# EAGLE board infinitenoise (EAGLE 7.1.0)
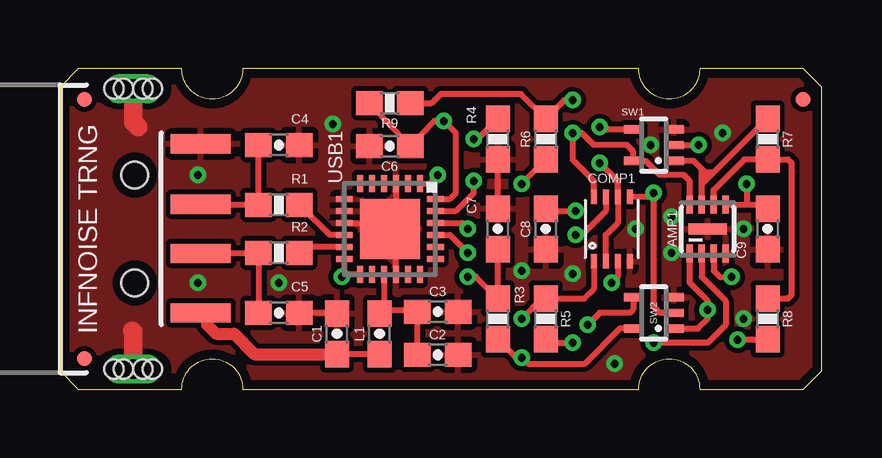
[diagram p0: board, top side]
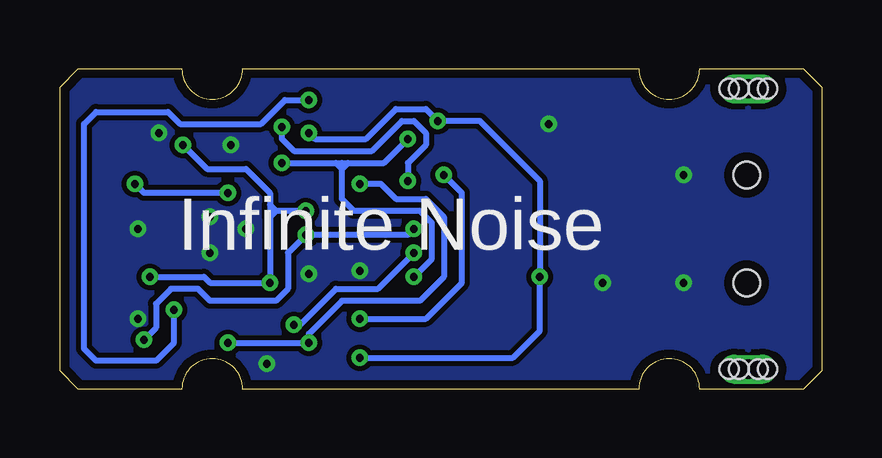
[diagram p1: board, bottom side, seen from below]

Size 31.75 x 13.36 mm. Coordinates in mm from the lower left corner, seen from the top.
Outline: 25.4,12.09 25.33,12.09
Outline: 25.4,12.09 arc90 26.67,13.36 30.99,13.36 31.75,12.6 31.75,0.76 30.99,0 26.67,0 arc90 25.4,1.27 arc90 24.13,0 7.62,0 arc90 6.35,1.27 arc90 5.08,0 0.76,0 0,0.76 0,12.6 0.76,13.36 5.08,13.36 arc90 6.35,12.09 arc90 7.62,13.36 24.13,13.36 arc90 25.4,12.09
Copper layers (1*16): Top 0.0356mm / dielectric 1.5011mm / Bottom 0.0356mm
Design rules "default *": minimum track width 8mil, minimum drill 13mil, track to track 8mil, track to pad 8mil, pad to pad 8mil, via to via 8mil, smd to smd 8mil, copper to edge 15mil, drill to drill 8mil, minimum pad ring 7mil, minimum via ring 7mil, stop-mask expansion 25mil, vias tented up to drill 14mil, thermal gap 10mil

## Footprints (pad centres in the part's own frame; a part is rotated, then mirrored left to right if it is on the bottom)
DFN6-2X3 = smd 0.28 x 0.75: 1 -0.75,-1.025; 2 -0.25,-1.025; 3 0.25,-1.025; 4 0.75,-1.025; 5 0.75,1.025; 6 0.25,1.025; 7 -0.25,1.025; 8 -0.75,1.025 | smd 1.6 x 0.45: EXP 0,0
0603-CAP = smd 1.1 x 1: 1 -0.85,0; 2 0.85,0
SSOP8-P-0.50A = smd 0.25 x 0.6: 1 -0.75,-1.35; 2 -0.25,-1.35; 3 0.25,-1.35; 4 0.75,-1.35; 5 0.75,1.35; 6 0.25,1.35; 7 -0.25,1.35; 8 -0.75,1.35
MICRO-FIDUCIAL = smd 0.635 x 0.635: 1 0,0
0603-IND = smd 1.1 x 1: 1 -0.85,0; 2 0.85,0
0603-RES = smd 1.1 x 1: 1 -0.85,0; 2 0.85,0
SC70-5L = smd 0.35 x 0.8: 1 -0.65,-0.85; 2 0,-0.85; 3 0.65,-0.85; 4 0.65,0.85; 5 -0.65,0.85
QFN24-4X4 = smd 0.7 x 0.25: 1 -1.9,1.25; 2 -1.9,0.75; 3 -1.9,0.25; 4 -1.9,-0.25; 5 -1.9,-0.75; 6 -1.9,-1.25; 13 1.9,-1.25; 14 1.9,-0.75; 15 1.9,-0.25; 16 1.9,0.25; 17 1.9,0.75; 18 1.9,1.25 | smd 0.25 x 0.7: 7 -1.25,-1.9; 8 -0.75,-1.9; 9 -0.25,-1.9; 10 0.25,-1.9; 11 0.75,-1.9; 12 1.25,-1.9; 19 1.25,1.9; 20 0.75,1.9; 21 0.25,1.9; 22 -0.25,1.9; 23 -0.75,1.9; 24 -1.25,1.9 | smd 2.5 x 2.5: EXP 0,0
USB-A-SMT-MALE = smd 0.8 x 2.5: 1 -3.5,-5.87; 2 -1.027,-5.87; 3 1.027,-5.87; 4 3.551,-5.87 | drill 0.8 pad 0.94 long: P$1 5.85,-3.05; P$3 -5.85,-3.05 | hole 1.1: 2.25,-3.12; -2.25,-3.12 | hole 0.8: -5.85,-3.45; -5.85,-3.85; -5.85,-2.65; -5.85,-2.25; 5.85,-3.45; 5.85,-3.85; 5.85,-2.65; 5.85,-2.25

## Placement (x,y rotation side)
AMP1  TSV912IQ2T  [DFN6-2X3]  27,6.68 0 top
C1  10nF  [0603-CAP]  11.55,2.31 90 top
C2  4.7uF  [0603-CAP]  15.75,1.43 0 top
C3  100nF  [0603-CAP]  15.75,3.23 0 top
C4  47pF  [0603-CAP]  9.12,10.18 0 top
C5  47pF  [0603-CAP]  9.12,3.18 0 top
C6  100nF  [0603-CAP]  13.75,10.13 180 top
C7  10nF  [0603-CAP]  18.25,6.68 90 top
C8  220pF  [0603-CAP]  20.25,6.68 90 top
C9  220pF  [0603-CAP]  29.5,6.68 90 top
COMP1  TC75W57FK  [SSOP8-P-0.50A]  23,6.68 0 top
FID1  FIDUCIALUFIDUCIAL  [MICRO-FIDUCIAL]  1.02,1.27 0 top
FID2  FIDUCIALUFIDUCIAL  [MICRO-FIDUCIAL]  1.02,12.09 0 top
FID3  FIDUCIALUFIDUCIAL  [MICRO-FIDUCIAL]  30.99,12.09 0 top
L1  FERRITE-BEAD0603-IND  [0603-IND]  13.32,2.31 90 top
R1  27  [0603-RES]  9.12,7.68 0 top
R2  27  [0603-RES]  9.12,5.68 0 top
R3  10K  [0603-RES]  18.25,2.93 90 top
R4  10K  [0603-RES]  18.25,10.43 90 top
R5  10K  [0603-RES]  20.25,2.93 270 top
R6  8.2K  [0603-RES]  20.25,10.43 90 top
R7  8.2K  [0603-RES]  29.5,10.43 270 top
R8  10K  [0603-RES]  29.5,2.93 270 top
R9  10K  [0603-RES]  13.75,11.93 180 top
SW1  MC74VHC1G66DFT1G  [SC70-5L]  24.75,10.18 90 top
SW2  MC74VHC1G66DFT1G  [SC70-5L]  24.75,3.18 90 top
USB1  FT240XQ  [QFN24-4X4]  13.75,6.68 270 top
X1  USBSMT-MALE  [USB-A-SMT-MALE]  0,6.68 90 top

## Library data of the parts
AMP1 C1-C9 COMP1 L1 R1-R9 SW1 SW2 USB1 X1 = infnoise
FID1-FID3 = SparkFun-Aesthetics

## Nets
A: AMP1.3 C8.2 COMP1.3 SW1.2
AMP1OUT: AMP1.1 R6.2 R9.1 SW2.1
AMP2OUT: AMP1.7 R7.1 SW1.1
B: AMP1.5 C9.2 COMP1.5 SW2.2
COMP1: COMP1.1 R5.1 USB1.1
COMP2: COMP1.7 R8.2 USB1.22
FB1: AMP1.2 R5.2 R6.1
FB2: AMP1.6 R7.2 R8.1
GND: AMP1.4 AMP1.EXP C1.2 C2.2 C3.2 C4.2 C5.2 C6.2 C7.2 C8.1 C9.1 COMP1.4 R4.1 SW1.3 SW2.3 USB1.3 USB1.7 USB1.8 USB1.9 USB1.16 USB1.EXP X1.4 X1.P$1 X1.P$3
N$2: R1.2 USB1.10
SW1EN: SW1.4 USB1.23
SW2EN: SW2.4 USB1.21
USB_M: C5.1 R2.1 X1.2
USB_P: C4.1 R1.1 X1.3
USBDM: R2.2 USB1.11
VCC: C2.1 C3.1 L1.2 USB1.15
VCC33: AMP1.8 C6.1 COMP1.8 R3.1 R9.2 SW1.5 SW2.5 USB1.12 USB1.13 USB1.24
VCCIN: C1.1 L1.1 X1.1
VREF: C7.1 COMP1.2 COMP1.6 R3.2 R4.2

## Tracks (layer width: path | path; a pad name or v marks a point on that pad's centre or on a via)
A  (via drill 0.33)
  Top 0.254: AMP1.3 27.25,4.93 27.5,4.68 v28,4.68 | SW1.2 v26.62,10.18 | COMP1.3 23.25,4.68 v23,4.43 | C8.2 20.35,7.43 v21.5,7.43
  Bottom 0.254: v26.62,10.18 25.62,9.18 24,9.18 23,8.18 23,7.68 | 23,7.68 23,7.43 | 23,7.43 23,7.18 | 23,7.18 v23,4.43 25.5,4.43 25.75,4.68 v28,4.68 | v21.5,7.43 22.75,7.43 | 22.75,7.43 23,7.43 | 22.75,7.43 23,7.68 | 22.75,7.43 23,7.18
AMP1OUT  (via drill 0.33)
  Top 0.254: SW2.1 26.6,2.53 27,2.93 v27,3.31 27,3.68 26.25,4.43 AMP1.1 | R9.1 15.5,11.93 15.88,12.3 19.23,12.3 R6.2 21.02,12.05 v21.38,12.05
  Bottom 0.254: v27,3.31 27,1.93 27.75,1.18 30.25,1.18 30.75,1.68 30.75,11.05 30.25,11.55 27.25,11.55 26.75,11.05 23.38,11.05 22.38,12.05 v21.38,12.05
AMP2OUT
  Top 0.254: AMP1.7 26.75,8.55 | 26.75,8.55 26.75,8.68 | 26.75,8.68 26.75,8.93 | 26.75,8.93 26.75,9.18 | 27.25,9.05 29.5,11.3 R7.1 | 27.25,9.05 27.12,8.93 | SW1.1 26.4,9.53 26.75,9.18 | 27.12,8.93 27,8.93 | 27,8.93 26.75,8.93 | 26.75,9.18 26.88,9.05 | 26.88,9.05 27,8.93 | 27,8.93 26.75,8.68 | 27.12,8.93 26.75,8.55 | 26.88,9.05 27.25,9.05
B  (via drill 0.33)
  Top 0.254: AMP1.5 28.62,7.71 | 28.62,7.71 29.32,7.71 C9.2 | COMP1.5 24.6,8.03 v24.75,8.18 24.75,3.43 25,3.18 SW2.2 | v28.62,8.55 28.62,7.71
  Bottom 0.254: v24.75,8.18 28.25,8.18 v28.62,8.55
COMP1  (via drill 0.33)
  Top 0.254: COMP1.1 22.25,4.18 21.85,3.78 R5.1 20.1,3.78 v19.25,2.93 | USB1.1 15.4,8.58 v15.75,8.93
  Bottom 0.254: v19.25,2.93 16.5,2.93 15,4.43 15,8.18 v15.75,8.93
COMP2  (via drill 0.33)
  Top 0.254: COMP1.7 22.75,7.43 21.75,6.43 v21.5,6.43 | USB1.22 16.75,6.93 v17,6.68 | R8.2 29.48,2.06 v28.25,2.06
  Bottom 0.254: v17,6.68 17.25,6.43 v21.5,6.43 22.25,5.68 22.25,4.18 22.75,3.68 25.5,3.68 26,4.18 27.12,4.18 27.75,3.56 27.75,2.56 v28.25,2.06
FB1  (via drill 0.33)
  Top 0.254: AMP1.2 26.75,4.68 27.75,3.68 27.75,2.68 27,1.93 v24.75,1.93 | R6.1 19.35,8.68 v19.25,8.55 | R5.2 20.52,1.93 v21.38,1.93 21.5,1.8
  Bottom 0.254: v19.25,8.55 18.38,8.55 17.75,7.93 16.5,7.93 15.75,7.18 15.75,4.68 16.75,3.68 20,3.68 21.38,2.31 v21.38,1.93 v24.75,1.93
FB2
  Top 0.254: AMP1.6 27.25,8.3 28.52,9.58 R7.2 30.35,9.58 30.5,9.43 30.5,3.93 30.35,3.78 R8.1
GND  (via drill 0.33)
  Top 0.254: USB1.16 14,6.43 USB1.EXP | USB1.3 14,6.93 USB1.EXP | C7.2 R4.1 | C1.2 11.35,3.18 C5.2 | USB1.9 13.5,6.93 USB1.EXP
  Top 0.762: X1.P$1 3.05,11.13 3.25,10.93 | X1.P$3 3.05,2.38 3,2.43
  other vias: 5.75,4.43 5.75,8.93 24,6.68 25.5,7.18 21.38,4.81 27.62,10.68 28.5,2.93 23.12,1.06 11.38,11.06 19.25,4.93 25.5,5.68 9.12,4.43 28.5,6.68 24.62,10.18
  pour Bottom: 0,13.43 0,-0.07 31.75,-0.07 31.75,13.43
  pour Top: 0,13.43 0,-0.07 31.75,-0.07 31.75,13.43
N$2
  Top 0.254: USB1.10 11.25,6.43 10.1,7.58 R1.2
SW1EN  (via drill 0.33)
  Top 0.254: USB1.23 16.5,7.43 17.25,8.18 v17.25,8.68 | SW1.4 22.6,10.83 v22.5,10.93
  Bottom 0.254: v17.25,8.68 17.25,9.43 16.5,10.18 16.5,10.68 17,11.18 17.5,11.18 18.75,9.93 22,9.93 22.5,10.43 v22.5,10.93
SW2EN  (via drill 0.33)
  Top 0.254: USB1.21 16.25,6.43 v17,5.68 | SW2.4 23.9,3.33 23.75,3.18 22.5,3.18 v22,2.68
  Bottom 0.254: v22,2.68 21.75,2.68 20.25,4.18 18.5,4.18 v17,5.68
USB_M
  Top 0.254: X1.2 5.9,5.68 R2.1 C5.1
USB_P
  Top 0.254: X1.3 8.37,7.71 | R1.1 C4.1
  Top 0.762: 8.37,7.71 R1.1
USBDM
  Top 0.254: USB1.11 10.35,5.93 R2.2
VCC
  Top 0.254: C2.1 C3.1 14.55,3.28 13.5,3.28 | 13.5,3.28 L1.2 | USB1.15 13.5,3.28
VCC33  (via drill 0.33)
  Top 0.254: R9.2 C6.1 15.6,11.18 v16,11.18 16.5,10.68 16.5,8.18 16.25,7.93 USB1.24 | USB1.12 11.85,4.78 | USB1.13 11.85,4.78 | 11.85,4.78 v11.75,4.68 | AMP1.8 26.25,8.68 26,8.93 25,8.93 24.4,9.53 SW1.5 23.9,9.9 23.62,10.18 22.25,10.18 21.75,10.68 v21.38,10.68 21.38,9.55 22.25,8.68 COMP1.8 | SW2.5 23.35,2.53 21.88,1.05 19.5,1.05 v19.25,1.3 19.02,1.3 R3.1
  Bottom 0.254: v19.25,1.3 12.88,1.3 11.75,2.43 v11.75,4.68 11.75,8.68 14.25,11.18 v16,11.18 16.5,11.68 17.75,11.68 19,10.43 21.12,10.43 v21.38,10.68
VCCIN
  Top 0.254: L1.1 C1.1
  Top 0.508: X1.1 6.12,2.92 6.12,2.68 6.5,2.31 7.25,2.31 8.1,1.46 C1.1
VREF  (via drill 0.33)
  Top 0.254: C7.1 R3.2 17.35,4.68 v17,4.68 | v22.5,9.43 23.25,8.68 COMP1.6 23.25,6.93 22.75,6.43 COMP1.2 | R4.2 17.4,10.43 v17.25,10.43
  Bottom 0.254: v17,4.68 16.25,5.43 16.25,6.93 16.75,7.43 19.5,7.43 20,7.93 20,9.18 | v22.5,9.43 20.25,9.43 | 20.25,9.43 20,9.43 | 20,9.43 19.75,9.43 | 19.75,9.43 18.25,9.43 v17.25,10.43 | 20,9.18 20,9.43 | 20,9.18 20.25,9.43 | 20,9.18 19.75,9.43

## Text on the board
tNames: INFNOISE TRNG
bNames: Infinite Noise

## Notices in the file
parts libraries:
SparkFun-Aesthetics: Licensing: Creative Commons ShareAlike 4.0 International - https://creativecommons.org/licenses/by-sa/4.0
